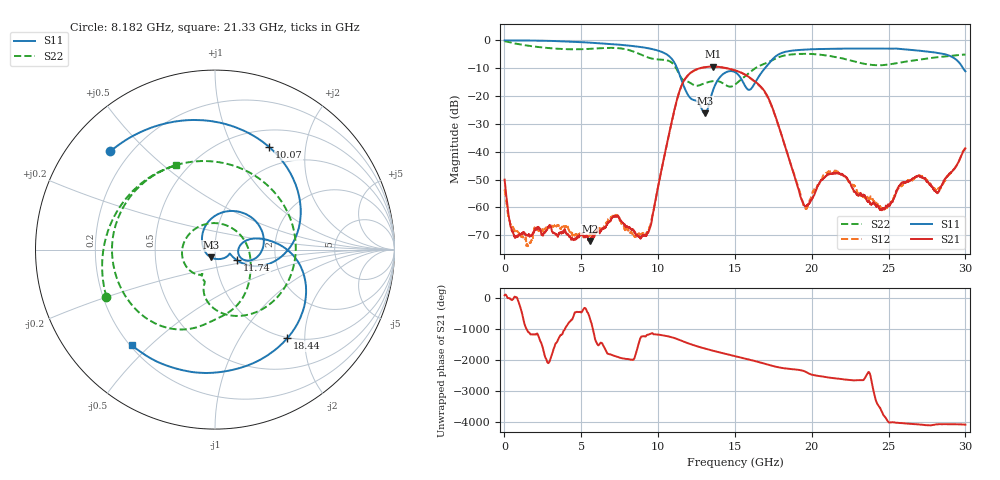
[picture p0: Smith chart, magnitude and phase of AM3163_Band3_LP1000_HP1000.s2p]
!Agilent Technologies,E8364B,MY43040894,A.07.50.67
!Agilent E8364B: A.07.50.67
!Date: Thursday, August 20, 2020 11:09:08
!Correction: S11(Full 2 Port(1,2))
!S21(Full 2 Port(1,2))
!S12(Full 2 Port(1,2))
!S22(Full 2 Port(1,2))
!S2P File: Measurements: S11, S21, S12, S22:
# Hz S  dB  R 50
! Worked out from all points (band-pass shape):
!   3201 points, 10 MHz to 30 GHz, reference 50 ohm
!   highest |S21| = -9.40 dB at 13.59 GHz (marker M1); lowest = -72.0 dB at 5.549 GHz (marker M2)
!   |S21| within 3 dB of the highest: 11.96 GHz to 15.69 GHz (3.728 GHz wide, 27 % of centre)
!   lowest |S11| = -26.2 dB at 13.05 GHz (marker M3), VSWR 1.10, Z = 47.5 - j4.03 ohm
!   |S11| at or under -10 dB: 11.24 GHz to 16.95 GHz (5.711 GHz wide, 40.5 % of centre); 29.85 GHz to end of sweep
!   |S22| runs from -16.6 to -0.3 dB; largest |S21 - S12| = 0.0058
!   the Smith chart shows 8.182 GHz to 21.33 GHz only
!   S11 on the Smith chart (normalised r, x): 8.182 GHz: 0.13, +0.39; 10.07 GHz: 0.72, +1.40; 11.74 GHz: 1.27, -0.15; 18.44 GHz: 0.99, -1.65; 21.33 GHz: 0.21, -0.44
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1e7  -0.03 -2.0  -50.03 84.2  -53.49 135.2  -0.29 -6.4
1.069022e9  -0.04 -29.1  -69.63 -8.1  -70.34 46.6  -1.51 -84.9
2.399828e9  -0.13 -65.2  -69.30 -12.0  -68.52 171.6  -2.51 -167.6
5.014581e9  -0.64 -134.1  -69.57 -103.5  -69.27 -11.1  -3.17 54.0
5.548778e9  -0.80 -148.2  -72.04 84.1  -70.05 24.6  -3.04 24.0
7.123253e9  -1.39 168.9  -63.10 -57.1  -62.66 -64.9  -2.71 -75.2
8.182275e9  -1.94 136.8  -67.46 178.3  -69.01 179.8  -3.61 -156.5
9.316272e9  -2.79 96.1  -68.93 -104.3  -68.37 -37.4  -6.09 96.1
1.000979e10  -3.69 65.0  -52.21 -97.2  -52.39 -100.9  -6.86 23.0
1.006602e10  -3.79 62.1  -50.77 -102.0  -50.72 -104.5  -6.88 17.1
1.174359e10  -17.38 -25.9  -13.92 19.0  -14.02 19.4  -14.53 -107.5
1.304628e10  -26.23 -119.8  -9.62 170.7  -9.68 171.0  -15.37 -125.8
1.358985e10  -17.68 117.9  -9.40 99.3  -9.51 99.5  -14.61 -150.5
1.5005e10  -11.40 3.6  -10.77 -71.8  -10.76 -71.3  -15.90 34.6
1.698247e10  -9.78 7.8  -18.75 36.0  -18.95 37.1  -8.28 -88.5
1.844448e10  -3.92 -50.7  -41.28 -119.2  -41.22 -115.5  -5.21 -140.2
1.953162e10  -3.34 -85.8  -59.51 159.9  -59.94 160.4  -4.83 -178.5
2.000958e10  -3.19 -98.8  -57.01 50.1  -55.37 50.4  -4.89 164.6
2.133102e10  -3.02 -131.0  -47.94 -55.8  -47.04 -52.8  -5.73 114.8
2.500479e10  -3.01 145.0  -58.97 -43.8  -59.15 -142.5  -8.68 -72.0
2.735713e10  -3.93 79.7  -49.45 -131.5  -49.66 -131.0  -6.65 -168.4
3e10  -11.10 -24.4  -38.78 -117.9  -38.66 -118.7  -5.10 108.7
